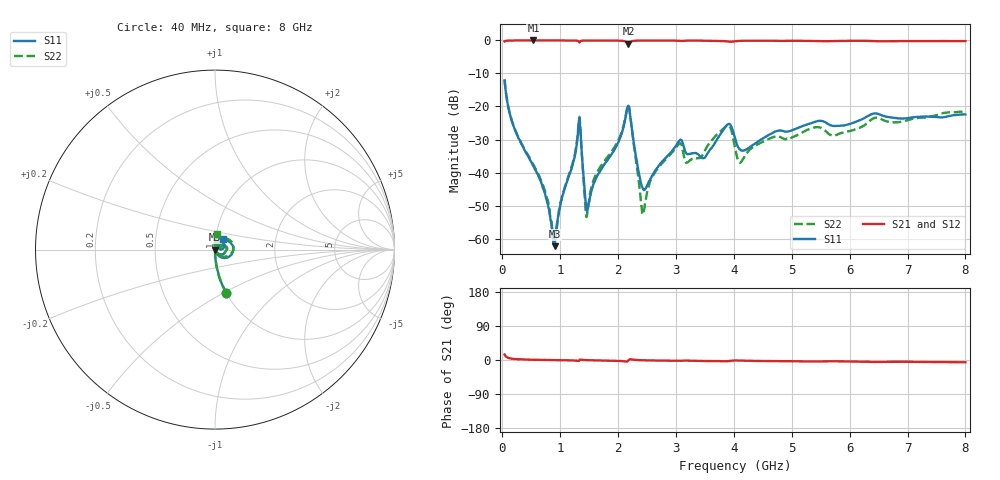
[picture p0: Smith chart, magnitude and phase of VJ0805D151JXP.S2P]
! VJ0805D151JXP
! DATE 03/14/2022  08:59
! CAPACITORS MOUNTED IN SERIES ON 25 MIL THICK MICROSTRIP SUBSTRATE
# GHz  S  MA  R  50.00
!  FREQ  S11M  S11A  S21M  S21A  S12M  S12A  S22M  S22A
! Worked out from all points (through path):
!   801 points, 40 MHz to 8 GHz, reference 50 ohm
!   highest |S21| = 0.00 dB at 537.5 MHz (marker M1); lowest = -0.9 dB at 2.179 GHz (marker M2)
!   lowest |S11| = -62.3 dB at 905.6 MHz (marker M3), VSWR 1.00, Z = 50.1 + j0.0219 ohm
!   |S11| at or under -10 dB: start of sweep to end of sweep
!   |S22| runs from -61.4 to -12.0 dB; largest |S21 - S12| = 0.0035
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0.04  0.2488 -75.4  0.9683 14.4  0.9667 14.4  0.2519 -75.8
0.1992  0.04925 -87.2  0.9985 2.8  0.9988 2.8  0.0498 -87.1
0.5375  0.01243 -88.1  0.9997 0.6  1 0.6  0.0131 -87.3
0.7564  0.004093 -82.7  0.9993 0.0  0.9998 0.0  0.00472 -81.9
0.90565  0.0007675 16.6  0.9991 -0.3  0.9993 -0.3  0.0009313 3.6
1.3136  0.04698 50.4  0.9717 -2.6  0.9718 -2.6  0.04933 53.4
1.3733  0.0196 -59.7  0.9897 0.6  0.9903 0.6  0.01963 -57.6
1.42305  0.005344 -50.0  0.9969 -0.2  0.9975 -0.2  0.004633 -48.3
1.4728  0.002724 17.1  0.9979 -0.5  0.9987 -0.5  0.002619 47.2
1.60215  0.007576 69.2  0.9984 -0.9  0.9988 -0.9  0.008742 81.9
2.17925  0.1027 -3.0  0.8969 -0.9  0.8974 -1.0  0.1048 6.5
2.428  0.005718 -17.1  0.9967 -0.7  0.9974 -0.8  0.002311 11.0
2.69665  0.01252 53.1  0.9967 -1.5  0.9978 -1.5  0.01197 85.0
3.07475  0.03144 34.5  0.9842 -2.2  0.9844 -2.2  0.02775 58.6
3.19415  0.01902 24.1  0.9939 -1.7  0.9945 -1.7  0.01419 61.5
3.49265  0.01679 49.5  0.9903 -2.7  0.9909 -2.8  0.02091 97.3
3.8807  0.05237 40.5  0.9656 -3.2  0.9669 -3.3  0.05142 57.5
4.02995  0.03086 2.0  0.9749 -1.3  0.9755 -1.3  0.02158 18.3
4.1195  0.02185 21.0  0.9868 -1.7  0.9875 -1.7  0.01434 58.6
5.3533  0.05644 47.5  0.9809 -3.9  0.9811 -4.0  0.04719 79.6
6.67665  0.06916 47.2  0.9728 -4.6  0.9734 -4.7  0.05871 69.4
8  0.07588 53.1  0.9773 -6.0  0.9778 -6.1  0.08534 81.8
